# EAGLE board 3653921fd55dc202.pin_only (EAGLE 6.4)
REV: B

Size 43.18 x 17.78 mm. Coordinates in mm from the lower left corner, seen from the top.
Outline: 0,15.75 0,11.68 0.25,11.43 0.25,6.6 0,6.35 0,2.03 arc90 2.03,0 41.15,0 arc90 43.18,2.03 43.18,15.75 arc90 41.15,17.78 2.03,17.78 arc90 0,15.75
Copper layers (1*16): Top 0.035mm / dielectric 1.5mm / Bottom 0.035mm
Design rules "adafruit *": minimum track width 8mil, minimum drill 15.5mil, track to track 8mil, track to pad 8mil, pad to pad 8mil, via to via 8mil, smd to smd 8mil, copper to edge 10mil, drill to drill 8mil, minimum pad ring 10mil, minimum via ring 8mil, stop-mask expansion 2mil, vias tented up to drill 20mil, thermal gap 10mil
Net classes: 1 power: width 0.305 mm, drill 0.483 mm, clearance 0.203 mm; 2 gnd: width 0.305 mm, drill 0.483 mm, clearance 0.203 mm; 3 usbvcc: width 0.305 mm, drill 0.483 mm, clearance 0.203 mm; 4 aref: width 0.254 mm, drill 0.483 mm, clearance 0.203 mm
Holes 2.2 mm at 1.91,15.88 1.91,1.91 41.27,15.88 41.02,1.91

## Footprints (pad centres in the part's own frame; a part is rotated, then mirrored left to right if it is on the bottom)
1X06_ROUND = drill 1 pad 1.676: 1 -6.35,0; 2 -3.81,0; 3 -1.27,0; 4 1.27,0; 5 3.81,0; 6 6.35,0
0805-NO = smd 1.3 x 1.5: 1 -0.95,0; 2 0.95,0
_0805MP = smd 1.2 x 1.3: 1 -1.016,0; 2 1.016,0
SOD-123 = smd 1.4 x 1.4: A 1.85,0; C -1.85,0
CHIPLED_0805_NOOUTLINE = smd 1.2 x 1.2: A 0,-1.05; C 0,1.05
FIDUCIAL_1MM = smd 1 x 1: 1 0,0
1X08_ROUND = drill 1 pad 1.676: 1 -8.89,0; 2 -6.35,0; 3 -3.81,0; 4 -1.27,0; 5 1.27,0; 6 3.81,0; 7 6.35,0; 8 8.89,0
1X08_ROUND_70 = drill 1 pad 1.778: 1 -8.89,0; 2 -6.35,0; 3 -3.81,0; 4 -1.27,0; 5 1.27,0; 6 3.81,0; 7 6.35,0; 8 8.89,0
RESPACK_4X0603 = smd 0.45 x 0.9: 1 -1.3,-0.85; 2 -0.4,-0.85; 3 0.4,-0.85; 4 1.3,-0.85; 5 1.3,0.85; 6 0.4,0.85; 7 -0.4,0.85; 8 -1.3,0.85
BTN_KMR2_4.6X2.8 = smd 0.9 x 1: A 2.05,0.8; A' -2.05,0.8; B 2.05,-0.8; B' -2.05,-0.8
SOT23-5 = smd 0.55 x 1.2: 1 -0.95,-1.3; 2 0,-1.3; 3 0.95,-1.3; 4 0.95,1.3; 5 -0.95,1.3
MLF32-TH = smd 0.7 x 0.25: 1 -2.35,1.75; 2 -2.35,1.25; 3 -2.35,0.75; 4 -2.35,0.25; 5 -2.35,-0.25; 6 -2.35,-0.75; 7 -2.35,-1.25; 8 -2.35,-1.75; 17 2.35,-1.75; 18 2.35,-1.25; 19 2.35,-0.75; 20 2.35,-0.25; 21 2.35,0.25; 22 2.35,0.75; 23 2.35,1.25; 24 2.35,1.75 | smd 0.25 x 0.7: 9 -1.75,-2.35; 10 -1.25,-2.35; 11 -0.75,-2.35; 12 -0.25,-2.35; 13 0.25,-2.35; 14 0.75,-2.35; 15 1.25,-2.35; 16 1.75,-2.35; 25 1.75,2.35; 26 1.25,2.35; 27 0.75,2.35; 28 0.25,2.35; 29 -0.25,2.35; 30 -0.75,2.35; 31 -1.25,2.35; 32 -1.75,2.35 | smd 3.2 x 3.2: TH 0,0
QFN24_4MM_SMSC = smd 0.8 x 0.28: 1 -2,1.25; 2 -2,0.75; 3 -2,0.25; 4 -2,-0.25; 5 -2,-0.75; 6 -2,-1.25; 13 2,-1.25; 14 2,-0.75; 15 2,-0.25; 16 2,0.25; 17 2,0.75; 18 2,1.25 | smd 0.28 x 0.8: 7 -1.25,-2; 8 -0.75,-2; 9 -0.25,-2; 10 0.25,-2; 11 0.75,-2; 12 1.25,-2; 19 1.25,2; 20 0.75,2; 21 0.25,2; 22 -0.25,2; 23 -0.75,2; 24 -1.25,2 | smd 2.5 x 2.5: THERM 0,0
SOLDERJUMPER_2WAY_OPEN_NOPASTE = smd 1.168 x 1.6: 1 -1.397,0; 2 0,0; 3 1.397,0
4UCONN_20329_V2 = smd 1 x 2: BASE@1 -0.75,-2; BASE@2 0.75,-2 | smd 0.4 x 1.35: D+ 0,0.775; D- -0.65,0.775; GND 1.3,0.775; ID 0.65,0.775; VBUS -1.3,0.775 | drill 0.8 pad 1.2 offset: SPRT@1 -3.3,0.9; SPRT@2 3.3,0.9 | drill 0.9 pad 2.5 square: SPRT@3 -3.6,-1.9; SPRT@4 3.6,-1.9 | hole 0.7: -1.95,0; 1.95,0
RESONATOR = smd 0.7 x 2: 1 -1,0; 2 0,0; 3 1,0

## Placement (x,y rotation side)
AD  20609  [1X06_ROUND]  31.75,1.27 0 top
AD1  20609  [1X06_ROUND]  11.43,16.51 180 top
C1  10uF  [0805-NO]  15.37,11.81 0 top
C2  10uF  [0805-NO]  17.65,5.08 270 top
C3  10uF  [0805-NO]  8.51,7.11 90 top
C4  0.1uF  [0805-NO]  29.15,4.93 0 top
C5  0.1uF  [_0805MP]  14.35,4.32 180 top
C6  0.1uF  [0805-NO]  20.45,8 180 top
C8  0.1uF  [0805-NO]  14.86,8 270 top
C10  0.1uF  [0805-NO]  37.27,11.6 135 top
C12  10uF  [0805-NO]  25.53,4.19 0 top
D3  MBR120  [SOD-123]  9.65,4.57 180 top
D4  YELLOW  [CHIPLED_0805_NOOUTLINE]  24.77,10.41 90 top
D5  YELLOW  [CHIPLED_0805_NOOUTLINE]  24.77,12.06 90 top
FD1  FIDUCIAL""  [FIDUCIAL_1MM]  7.11,13.34 0 top
FD2  FIDUCIAL""  [FIDUCIAL_1MM]  40.89,8.89 0 top
IOL  20610  [1X08_ROUND]  29.21,16.51 0 top
L  RED  [CHIPLED_0805_NOOUTLINE]  24.64,7.11 90 top
ON  GREEN  [CHIPLED_0805_NOOUTLINE]  24.64,8.76 90 top
POWER1  20610  [1X08_ROUND_70]  13.97,1.27 0 top
R2  1K  [RESPACK_4X0603]  20.95,11.05 270 top
R8  10K  [0805-NO]  40.39,12.45 0 top
R11  1K  [0805-NO]  38.1,5.46 270 top
RESET  KMR2  [BTN_KMR2_4.6X2.8]  40.89,8.89 270 top
U1  MIC5225-5.0  [SOT23-5]  20.7,5.33 90 top
U2  ATMEGA328P  [MLF32-TH]  33.02,8.51 225 top
U3  CP2104  [QFN24_4MM_SMSC]  10.92,11.43 0 top
U4  MIC5225-3.3  [SOT23-5]  11.68,7.11 270 top
U$4  [PCBFEAT-REV-040]  17.02,8.64 0 top
U$5  [ADAFRUIT_2.5MM]  28.57,10.41 0 top
U$7  [METROMINI_SILK]  42.93,2.54 0 bottom
U$10  [ADAFRUIT_5MM]  42.55,9.91 0 bottom
U$12  [SYMBOL_CE_TINY]  11.68,9.53 0 bottom
U$14  [SYMBOL_FCC_TINY]  16.38,9.65 0 bottom
VSELECT  [SOLDERJUMPER_2WAY_OPEN_NOPASTE]  11.81,5.84 180 bottom
X1  20329  [4UCONN_20329_V2]  4.32,8.89 270 top
Y2  CSTCE16M0V53-R0 16MHZ  [RESONATOR]  33.8,13.21 0 top

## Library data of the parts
AD AD1 C1-C6 C8 C10 C12 D3-D5 IOL L ON POWER1 R2 R8 R11 RESET U1-U4 U$4 U$5 U$7 U$10 U$12 U$14 VSELECT X1 = microbuilder
FD1 FD2 = microbuilder; BOM: EXCLUDE
Y2 = SmartPrj

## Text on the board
tPlace: 13 | 12 | 11 | 10 | 9 | 8 | 7 | 6 | 5 | 4 | 3 | 2 | 1 | 0 | Metro Mini | TX | CP2104 | RX | ON | Aref | RST | USB | Rst | 3V | 5V | GND | Vin | A0 | A1 | A2 | A3 | A4 | A5
bPlace: ATmega328 @16MHz | Vin:5-16VDC | 3v | 5v | Vio
tNames: IOREF | RESET | 3V3 | 5V | GND | VIN
ReferenceLC: PC1 | PC2
214bmp: D:/SmartProjects/Snc/a4_bn_logo2.bmp

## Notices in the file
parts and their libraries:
microbuilder: This work is placed in the public domain, and may be freely used for commercial and non-commercial work with the following conditions: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
